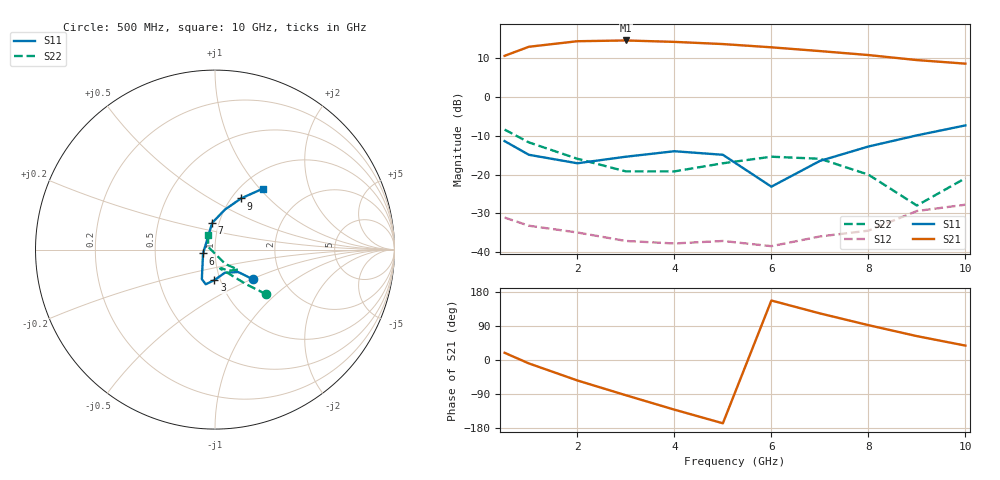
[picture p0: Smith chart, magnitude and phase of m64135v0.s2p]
!  MGA-64135 S PARAMETERS
!  Vd=10V  LAST UPDATED 07-22-92
# ghz s ma r 50
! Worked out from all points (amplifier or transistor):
!   11 points, 500 MHz to 10 GHz, reference 50 ohm
!   highest |S21| = 14.5 dB at 3 GHz (marker M1)
!   |S21| within 3 dB of that: 705.2 MHz to 7.26 GHz (6.555 GHz wide, 165 % of centre)
!   unconditionally stable (mu >= 1): start of sweep to end of sweep
!   at 1 GHz: K = 4.67, MAG = 13.4 dB, |S12| = -33.2 dB
!   at 5 GHz: K = 7.08, MAG = 13.9 dB, |S12| = -37.1 dB
!   at 10 GHz: K = 3.76, MAG = 9.5 dB, |S12| = -27.7 dB
!   S11 on the Smith chart (normalised r, x): 500 MHz: 1.43, -0.51; 3 GHz: 0.94, -0.33; 6 GHz: 0.87, -0.04; 7 GHz: 0.93, +0.28; 9 GHz: 1.11, +0.70; 10 GHz: 1.24, +1.03
0.5  0.27 -38.0  3.38 19.0  0.028 -13.0  0.38 -41.0
1  0.18 -44.0  4.42 -9.0  0.022 -20.0  0.26 -48.0
2  0.14 -67.0  5.21 -54.0  0.018 -19.0  0.16 -59.0
3  0.17 -91.0  5.33 -93.0  0.014 -21.0  0.11 -75.0
4  0.2 -105.0  5.11 -131.0  0.013 -15.0  0.11 -71.0
5  0.18 -114.0  4.79 -167.0  0.014 -10.0  0.14 -57.0
6  0.07 -162.0  4.35 157.0  0.012 -1.0  0.17 -41.0
7  0.15 96.0  3.89 123.0  0.016 3.0  0.16 -42.0
8  0.23 76.0  3.46 92.0  0.019 4.0  0.1 -54.0
9  0.32 63.0  2.98 63.0  0.034 12.0  0.04 159.0
10  0.43 52.0  2.68 38.0  0.041 -11.0  0.09 116.0
